TYPE dut_PMC_to_PLC :
STRUCT
	bHeartBeatMonitor	: BOOL;		

	// UI switch
	DP_sw						,
	BWR_sw						,
	DPR1_sw						,
	DPR2_sw						,
	WAT_R_sw					,
	WAT_F_sw					,
	HTR1_sw						,
	HTR2_sw						,
	HTR3_sw						,
	HTR4_sw						,
	HTR5_sw						,
	AGV_sw						,
	DEPO_sw						,
	CLN_sw						,
	T_MNT_sw					,
	T_REF_sw					,
	Pump1_ECO_sw				,
	SP1_sw						,
	PZ_sw						,
	P_CONT_sw					,
	DGZERO_sw					,
	C_EXH_sw					,
	F2_CLN_sw					,
	F_N_sw						,
	GV_AV79_Open				,
	GV_AV79_Close				,
	APC_AV71_Open				,
	APC_AV71_Close				
	: BOOL;
	
	aAV							: ARRAY[1..250] OF BOOL;	
	bAV65Open					: BOOL;
	bAV65Close					: BOOL;
	bAV79Open					: BOOL;
	bAV79Close					: BOOL;
	bAV91Open					: BOOL;
	bAV91Close					: BOOL;
	bAV202Open					: BOOL;
	bAV202Close					: BOOL;
	
	//heater
	Furnace_Temp_abnormal		: BOOL;	// Furnace temp over 1000℃
	LSC_Ht_temp_abnormal		: BOOL;	// LSC heater temperature beyond preset value
	GB_Ht_temp_abnormal			: BOOL; // Gas line heater temperature beyond preset value
	EXH_Ht_temp_abnormal		: BOOL;	// Exhaust line heater temperature beyond preset value
	CLN_Temp_abnormal			: BOOL; // furnace&exhaust line heater temperature beyond preset value
	R_Axis_Temp					: REAL;	// R axis temperature
	Inlet_Ht_1_temp				: REAL;	// Inlet heater 1 temperature
	Inlet_Ht_2_temp				: REAL;	// Inlet heater 2 temperature
	Port_Ht_1_temp				: REAL; // Port heater 1 temperature
	Port_Ht_2_temp				: REAL; // Port heater 2 temperature
	Port_Ht_3_temp				: REAL; // Port heater 3 temperature
	Port_Ht_4_temp				: REAL; // Port heater 4 temperature
	Port_Ht_5_temp				: REAL; // Port heater 5 temperature

	//Power box
	I100_00			:BOOL;	//	UPS_Fault              
	I100_01			:BOOL;	//	UPS_Alarm              
	I100_02			:BOOL;	//	UPS_Bypass_Status      
	I100_03			:BOOL;	//	UPS_Battery_Voltage_Low
	I100_04			:BOOL;	//	UPS_Start              
	I100_05			:BOOL;	//	UPS_AC_Input_Cut_Off   
	I100_06			:BOOL;	//	Powerbox_FrontDoor_sw1
	I100_07			:BOOL;	//	Powerbox_FrontDoor_sw2
	I100_08			:BOOL;	//	Powerbox_BackDoor_sw1
	I100_09			:BOOL;	//	Powerbox_BackDoor_sw2
	I100_10			:BOOL;	//	Spare11
	I100_11			:BOOL;	//	Spare12
	I100_12			:BOOL;	//	Spare13
	I100_13			:BOOL;	//	Spare14
	I100_14			:BOOL;	//	Spare15
	I100_15			:BOOL;	//	Spare16
	I101_00			:BOOL;	//	KM101_ON
	I101_01			:BOOL;	//	KM201_ON
	I101_02			:BOOL;	//	KM102_ON
	I101_03			:BOOL;	//	KM103_ON
	I101_04			:BOOL;	//	KM104_ON
	I101_05			:BOOL;	//	SPARE
	I101_06			:BOOL;	//	SPARE
	I101_07			:BOOL;	//	Furnace_Main_Breaker_Status_Monitor
	I101_08			:BOOL;	//	Blower_Breaker_Status_Feedback
	I101_09			:BOOL;	//	Zone1_Circuit_Breaker_Status_Monitor
	I101_10			:BOOL;	//	Zone2_Circuit_Breaker_Status_Monitor
	I101_11			:BOOL;	//	Zone3_Circuit_Breaker_Status_Monitor
	I101_12			:BOOL;	//	Zone4_Circuit_Breaker_Status_Monitor
	I101_13			:BOOL;	//	Zone5_Circuit_Breaker_Status_Monitor
	I101_14			:BOOL;	//	Zone6_Circuit_Breaker_Status_Monitor
	I101_15			:BOOL;	//	Zone7_Circuit_Breaker_Status_Monitor
	I102_00			:BOOL;	//	LDS1_bulk_to_process_running
	I102_01			:BOOL;	//	LDS1_supply_doing
	I102_02			:BOOL;	//	LDS1_system_ready
	I102_03			:BOOL;	//	LDS1_major_alarm
	I102_04			:BOOL;	//	LDS1_minor_alarm
	I102_05			:BOOL;	//	LDS1_low_level_status
	I102_06			:BOOL;	//	LDS1_process_reservoir_empty
	I102_07			:BOOL;	//	LDS2_bulk_to_process_running
	I102_08			:BOOL;	//	LDS2_supply_doing           
	I102_09			:BOOL;	//	LDS2_system_ready           
	I102_10			:BOOL;	//	LDS2_major_alarm            
	I102_11			:BOOL;	//	LDS2_minor_alarm            
	I102_12			:BOOL;	//	LDS2_low_level_status       
	I102_13			:BOOL;	//	LDS2_process_reservoir_empty
	I102_14			:BOOL;	//	SPARE
	I102_15			:BOOL;	//	SPARE
	I103_00			:BOOL;	//	Vaccum1_Pump_Both_On
	I103_01			:BOOL;	//	Vaccum1_Pump_Warning
	I103_02			:BOOL;	//	Vaccum1_Pump_Alarm
	I103_03			:BOOL;	//	Spare19
	I103_04			:BOOL;	//	Spare20
	I103_05			:BOOL;	//	Spare21
	I103_06			:BOOL;	//	N2_Purge_BOX_PG13_CNT1
	I103_07			:BOOL;	//	N2_Purge_BOX_PG13_CNT2
	I103_08			:BOOL;	//	N2_Purge_BOX_PG14_CNT1
	I103_09			:BOOL;	//	N2_Purge_BOX_PG14_CNT2
	I103_10			:BOOL;	//	N2_Purge_Box_PG15_CNT1
	I103_11			:BOOL;	//	N2_Purge_Box_PG15_CNT2
	I103_12			:BOOL;	//	N2_Purge_Box_PG16_CNT1
	I103_13			:BOOL;	//	N2_Purge_Box_PG16_CNT2
	I103_14			:BOOL;	//	N2_Purge_Box_PG130_CNT1
	I103_15			:BOOL;	//	N2_Purge_Box_PG130_CNT2
	I104_00			:BOOL;	//	PS17_Low_pressure_alarm
	I104_01			:BOOL;	//	Foreline_heater_light_alarm
	I104_02			:BOOL;  //	Foreline_heater_heavy_alarm
	I104_03			:BOOL;  //	Scrubber_warning
	I104_04			:BOOL;  //	Scrubber_alarm
	I104_05			:BOOL;  //	External_HPM_alarm
	I104_06			:BOOL;  //	External_EMO_In
	I104_07			:BOOL;  //	SPARE
	I104_08			:BOOL;  //	SPARE
	I104_09			:BOOL;  //	SPARE
	I104_10			:BOOL;  //	SPARE
	I104_11			:BOOL;  //	SPARE
	I104_12			:BOOL;  //	SPARE
	I104_13			:BOOL;  //	SPARE
	I104_14			:BOOL;  //	SPARE
	I104_15			:BOOL;  //	SPARE
	
	Q100_00			:BOOL;	//	VFD_RES
	Q100_01			:BOOL;	//	VFD_MRS
	Q100_02			:BOOL;	//	VFD_RT
	Q100_03			:BOOL;	//	VFD_JOG
	Q100_04			:BOOL;	//	VFD_RL
	Q100_05			:BOOL;	//	VFD_RM
	Q100_06			:BOOL;	//	VFD_RH
	Q100_07			:BOOL;	//	VFD_STP
	Q100_08			:BOOL;	//	VFD_RTR
	Q100_09			:BOOL;	//	VFD_RTF
	Q100_10			:BOOL;	//	Spare1
	Q100_11			:BOOL;	//	Spare2
	Q100_12			:BOOL;	//	Spare3
	Q100_13			:BOOL;	//	Spare4
	Q100_14			:BOOL;	//	Spare5
	Q100_15			:BOOL;	//	Spare6
	Q101_00			:BOOL;	//	Furnace 1 Zone Heating Enable
	Q101_01			:BOOL;	//	Furnace 2 Zone Heating Enable
	Q101_02			:BOOL;	//	Furnace 3 Zone Heating Enable
	Q101_03			:BOOL;	//	Furnace 4 Zone Heating Enable
	Q101_04			:BOOL;	//	Furnace 5 Zone Heating Enable
	Q101_05			:BOOL;	//	Furnace 6 Zone Heating Enable
	Q101_06			:BOOL;	//	Furnace 7 Zone Heating Enable
	Q101_07			:BOOL;	//	LSC_1_AutoRefill1 Request Or Valve Open
	Q101_08			:BOOL;	//	LSC_1_External_Shutdown
	Q101_09			:BOOL;	//	HPM Valve Out Status
	Q101_10			:BOOL;	//	Forline Heater On
	Q101_11			:BOOL;	//	Spare7
	Q101_12			:BOOL;	//	Spare8
	Q101_13			:BOOL;	//	Spare9
	Q101_14			:BOOL;	//	Spare10
	Q101_15			:BOOL;	//	Spare11
	Q102_00			:BOOL;	//	Vaccum Pump Both On
	Q102_01			:BOOL;	//	Vaccum Pump AUC On
	Q102_02			:BOOL;	//	Vaccum Pump AGV Open
	Q102_03			:BOOL;	//	LSC_2_AutoRefill1 Request Or Valve Open
	Q102_04			:BOOL;	//	LSC_2_External_Shutdown
	Q102_05			:BOOL;	//	Spare
	Q102_06			:BOOL;	//	Spare
	Q102_07			:BOOL;	//	Spare
	Q102_08			:BOOL;	//	Spare
	Q102_09			:BOOL;	//	Spare
	Q102_10			:BOOL;	//	Spare
	Q102_11			:BOOL;	//	Spare
	Q102_12			:BOOL;	//	Spare
	Q102_13			:BOOL;	//	Spare
	Q102_14			:BOOL;	//	Spare
	Q102_15			:BOOL;	//	Spare
	Q103_00			:BOOL;	//	Spare
	Q103_01			:BOOL;	//	Spare
	Q103_02			:BOOL;	//	Spare
	Q103_03			:BOOL;	//	Spare
	Q103_04			:BOOL;	//	Spare
	Q103_05			:BOOL;	//	Spare
	Q103_06			:BOOL;	//	Spare
	Q103_07			:BOOL;	//	Spare
	Q103_08			:BOOL;	//	Spare
	Q103_09			:BOOL;	//	Spare
	Q103_10			:BOOL;	//	Spare
	Q103_11			:BOOL;	//	Spare
	Q103_12			:BOOL;	//	Spare
	Q103_13			:BOOL;	//	Spare
	Q103_14			:BOOL;	//	Spare
	Q103_15			:BOOL;	//	Spare	
	
	PS17_Pressure				: REAL;	// PS17_Pressure
	
	//Gas box
	Q200_00			:BOOL;	//	OX_Pump_On
	Q200_01			:BOOL;	//	Spare1
	Q200_02			:BOOL;	//	Spare2
	Q200_03			:BOOL;	//	Spare3
	Q200_04			:BOOL;	//	Spare4
	Q200_05			:BOOL;	//	Spare5
	Q200_06			:BOOL;	//	Spare6
	Q200_07			:BOOL;	//	Spare7
	Q200_08			:BOOL;	//	Spare8
	Q200_09			:BOOL;	//	Spare9
	Q200_10			:BOOL;	//	Spare10
	Q200_11			:BOOL;	//	Spare11
	Q200_12			:BOOL;	//	Spare12
	Q200_13			:BOOL;	//	Spare13
	Q200_14			:BOOL;	//	Spare14
	Q200_15			:BOOL;	//	Spare15
	
	VG31_Reading_Valid					: BOOL;
	VG31_Overrange_Exceeded				: BOOL;
	VG31_Underrange_Exceeded			: BOOL;
	VG31_Sensor_Value					: REAL;	
	VG31_Active_Device_Warning_Details	: UDINT;
	VG31_Active_Device_Error_Details	: UDINT;
	
	//Exhaust box
	Q300_00				:BOOL;	//	CoolingValve1_Boat
	Q300_01				:BOOL;	//	CoolingValve2_Flange
	Q300_02				:BOOL;
	Q300_03				:BOOL;
	Q300_04				:BOOL;
	Q300_05				:BOOL;
	Q300_06				:BOOL;
	Q300_07				:BOOL;
	Q300_08				:BOOL;	//	APC_auto_close
	Q300_09				:BOOL;	//	APC_pump_on
	Q300_10				:BOOL;	//	BallValve_Open_Close
	Q300_11				:BOOL;
	Q300_12				:BOOL;
	Q300_13				:BOOL;
	Q300_14				:BOOL;
	Q300_15				:BOOL;

	VG11_Reading_Valid					: BOOL;
	VG11_Overrange_Exceeded				: BOOL;
	VG11_Underrange_Exceeded			: BOOL;
	VG11_Sensor_Value					: REAL;	
	VG11_Active_Device_Warning_Details	: UDINT;
	VG11_Active_Device_Error_Details	: UDINT;
	
	VG13_Reading_Valid					: BOOL;
	VG13_Overrange_Exceeded				: BOOL;
	VG13_Underrange_Exceeded			: BOOL;
	VG13_Sensor_Value					: REAL;	
	VG13_Active_Device_Warning_Details	: UDINT;
	VG13_Active_Device_Error_Details	: UDINT;
	
	VG14_Reading_Valid					: BOOL;
	VG14_Overrange_Exceeded				: BOOL;
	VG14_Underrange_Exceeded			: BOOL;
	VG14_Sensor_Value					: REAL;	
	VG14_Active_Device_Warning_Details	: UDINT;
	VG14_Active_Device_Error_Details	: UDINT;
	
	//Frontbody box
	FB_Buffer_N2_Press_Low		: BOOL;
	
	//LA box
	LA_Buffer_N2_Press_Low		: BOOL;
	Boat_at_cap_position		: BOOL;
	
	I500_00			:BOOL;	//	FIMS1_FOUP_Dock
	I500_01			:BOOL;	//	FIMS1_FOUP_Undock
	I500_02			:BOOL;	//	FIMS1_FOUP_Exist
	I500_03			:BOOL;	//	FIMS2_FOUP_Dock
	I500_04			:BOOL;	//	FIMS2_FOUP_Undock
	I500_05			:BOOL;	//	FIMS2_FOUP_Exist
	I500_06			:BOOL;	//	FIMS1_FOUP_Wafer_Shift_Detection
	I500_07			:BOOL;	//	FIMS2_FOUP_Wafer_Shift_Detection
	I500_08			:BOOL;	//	FIMS1_FOUP_Negative_Pressure
	I500_09			:BOOL;	//	FIMS1_FOUP_Ordinary_Pressure
	I500_10			:BOOL;	//	FIMS2_FOUP_Negative_Pressure
	I500_11			:BOOL;	//	FIMS2_FOUP_Ordinary_Pressure
	I500_12			:BOOL;	//	BOAT_Slow_Down_Position_Detection
	I500_13			:BOOL;	//	Buffer_Rotation_Conv_Detect_Sensor
	I500_14			:BOOL;	//	Spare1
	I500_15			:BOOL;	//	Spare2
	I501_00			:BOOL;	//	LA_Internal_Cycle_Switch_Open
	I501_01			:BOOL;	//	LA_Internal_Cycle_Switch_Close
	I501_02			:BOOL;	//	LA_ATM_Switch_Open
	I501_03			:BOOL;	//	LA_ATM_Switch_Close
	I501_04			:BOOL;	//	R-Axis_Air_Cylinder_Extend_Position
	I501_05			:BOOL;	//	R-Axis_Air_Cylinder_Retract_Position
	I501_06			:BOOL;	//	Furnace_Shutter_Open
	I501_07			:BOOL;	//	Furnace_Shutter_Close
	I501_08			:BOOL;	//	FIMS1_Exhaust_Open_Position
	I501_09			:BOOL;	//	FIMS1_Exhaust_Close_Position
	I501_10			:BOOL;	//	FIMS2_Exhaust_Open_Position
	I501_11			:BOOL;	//	FIMS2_Exhaust_Close_Position
	I501_12			:BOOL;	//	Spare3
	I501_13			:BOOL;	//	Spare4
	I501_14			:BOOL;	//	Spare5
	I501_15			:BOOL;	//	Spare6
	I502_00			:BOOL;	//	FIMS1_Seal
	I502_01			:BOOL;	//	FIMS1_Release
	I502_02			:BOOL;	//	FIMS1_Door_Close
	I502_03			:BOOL;	//	FIMS1_Door_Open
	I502_04			:BOOL;	//	FIMS1_FOUP_Latch_Off
	I502_05			:BOOL;	//	FIMS1_FOUP_Latch_On
	I502_06			:BOOL;	//	FIMS1_Collision_Avoidance_Up
	I502_07			:BOOL;	//	FIMS1_Collision_Avoidance_Down
	I502_08			:BOOL;	//	FIMS2_Seal
	I502_09			:BOOL;	//	FIMS2_Release
	I502_10			:BOOL;	//	FIMS2_Door_Close
	I502_11			:BOOL;	//	FIMS2_Door_Open
	I502_12			:BOOL;	//	FIMS2_FOUP_Latch_Off
	I502_13			:BOOL;	//	FIMS2_FOUP_Latch_On
	I502_14			:BOOL;	//	FIMS2_Collision_Avoidance_Up
	I502_15			:BOOL;	//	FIMS2_Collision_Avoidance_Down
	I503_00			:BOOL;	//	Spare7
	I503_01			:BOOL;	//	Spare8
	I503_02			:BOOL;	//	Spare9
	I503_03			:BOOL;	//	Spare10
	I503_04			:BOOL;	//	Spare11
	I503_05			:BOOL;	//	Spare12
	I503_06			:BOOL;	//	Spare13
	I503_07			:BOOL;	//	Spare14
	I503_08			:BOOL;	//	Spare15
	I503_09			:BOOL;	//	Spare16
	I503_10			:BOOL;	//	Spare17
	I503_11			:BOOL;	//	Spare18
	I503_12			:BOOL;	//	Spare19
	I503_13			:BOOL;	//	Spare20
	I503_14			:BOOL;	//	Spare21
	I503_15			:BOOL;	//	Spare22
	I504_00			:BOOL;	//	Spare23
	I504_01			:BOOL;	//	Spare24
	I504_02			:BOOL;	//	Spare25
	I504_03			:BOOL;	//	Spare26
	I504_04			:BOOL;	//	Spare27
	I504_05			:BOOL;	//	Spare28
	I504_06			:BOOL;	//	Spare29
	I504_07			:BOOL;	//	Spare30
	I504_08			:BOOL;	//	Spare31
	I504_09			:BOOL;	//	Spare32
	I504_10			:BOOL;	//	Spare33
	I504_11			:BOOL;	//	Spare34
	I504_12			:BOOL;	//	Spare35
	I504_13			:BOOL;	//	Spare36
	I504_14			:BOOL;	//	Spare37
	I504_15			:BOOL;	//	Spare38
	I505_00			:BOOL;	//	Buffer_A1_N2_Pressure_Alarm
	I505_01			:BOOL;	//	Buffer_A1_FOUP_Detect
	I505_02			:BOOL;	//	Buffer_B1_N2_Pressure_Alarm
	I505_03			:BOOL;	//	Buffer_B1_FOUP_Detect
	I505_04			:BOOL;	//	Buffer_C1_N2_Pressure_Alarm
	I505_05			:BOOL;	//	Buffer_C1_FOUP_Detect
	I505_06			:BOOL;	//	Buffer_D1_N2_Pressure_Alarm
	I505_07			:BOOL;	//	Buffer_D1_FOUP_Detect
	I505_08			:BOOL;	//	Buffer_A2_N2_Pressure_Alarm
	I505_09			:BOOL;	//	Buffer_A2_FOUP_Detect
	I505_10			:BOOL;	//	Buffer_B2_N2_Pressure_Alarm
	I505_11			:BOOL;	//	Buffer_B2_FOUP_Detect
	I505_12			:BOOL;	//	Buffer_C2_N2_Pressure_Alarm
	I505_13			:BOOL;	//	Buffer_C2_FOUP_Detect
	I505_14			:BOOL;	//	Buffer_D2_N2_Pressure_Alarm
	I505_15			:BOOL;	//	Buffer_D2_FOUP_Detect
	I506_00			:BOOL;	//	Buffer_A3_N2_Pressure_Alarm
	I506_01			:BOOL;	//	Buffer_A3_FOUP_Detect
	I506_02			:BOOL;	//	Buffer_B3_N2_Pressure_Alarm
	I506_03			:BOOL;	//	Buffer_B3_FOUP_Detect
	I506_04			:BOOL;	//	Buffer_C3_N2_Pressure_Alarm
	I506_05			:BOOL;	//	Buffer_C3_FOUP_Detect
	I506_06			:BOOL;	//	Buffer_D3_N2_Pressure_Alarm
	I506_07			:BOOL;	//	Buffer_D3_FOUP_Detect
	I506_08			:BOOL;	//	Buffer_A4_N2_Pressure_Alarm
	I506_09			:BOOL;	//	Buffer_A4_FOUP_Detect
	I506_10			:BOOL;	//	Buffer_B4_N2_Pressure_Alarm
	I506_11			:BOOL;	//	Buffer_B4_FOUP_Detect
	I506_12			:BOOL;	//	Buffer_C4_N2_Pressure_Alarm
	I506_13			:BOOL;	//	Buffer_C4_FOUP_Detect
	I506_14			:BOOL;	//	Buffer_D4_N2_Pressure_Alarm
	I506_15			:BOOL;	//	Buffer_D4_FOUP_Detect
	
	Q500_00			:BOOL;	//	LA_Internal_Air_Cycle_Switch_Open
	Q500_01			:BOOL;	//	LA_Internal_Air_Cycle_Switch_Close
	Q500_02			:BOOL;	//	LA_ATM_Switch_Open
	Q500_03			:BOOL;	//	LA_ATM_Switch_Close
	Q500_04			:BOOL;	//	R_Axis_Air_Cylinder_Extend_Switch
	Q500_05			:BOOL;	//	R_Axis_Air_Cylinder_Retract_Switch
	Q500_06			:BOOL;	//	O2_Detector_Switch_LA_POD
	Q500_07			:BOOL;	//	O2_Detector_Switch_POD1_POD2
	Q500_08			:BOOL;	//	LA_Internal_Air_Cycle_Fan1_Switch
	Q500_09			:BOOL;	//	LA_Internal_Air_Cycle_Fan2_Switch
	Q500_10			:BOOL;	//	LA_Internal_Air_Cycle_Fan3_Switch
	Q500_11			:BOOL;	//	LA_Internal_Air_Cycle_Fan4_Switch
	Q500_12			:BOOL;	//	Furnace_Shutter_Open
	Q500_13			:BOOL;	//	Furnace_Shutter_Close
	Q500_14			:BOOL;	//	Spare1
	Q500_15			:BOOL;	//	Spare2
	Q501_00			:BOOL;	//	POD1_Exhaust_Switch_Open
	Q501_01			:BOOL;	//	POD1_Exhaust_Switch_Close
	Q501_02			:BOOL;	//	POD2_Exhaust_Switch_Open
	Q501_03			:BOOL;	//	POD2_Exhaust_Switch_Close
	Q501_04			:BOOL;	//	Spare3
	Q501_05			:BOOL;	//	Spare4
	Q501_06			:BOOL;	//	Spare5
	Q501_07			:BOOL;	//	Spare6
	Q501_08			:BOOL;	//	Spare7
	Q501_09			:BOOL;	//	Spare8
	Q501_10			:BOOL;	//	Spare9
	Q501_11			:BOOL;	//	Spare10
	Q501_12			:BOOL;	//	Spare11
	Q501_13			:BOOL;	//	Spare12
	Q501_14			:BOOL;	//	Spare13
	Q501_15			:BOOL;	//	Spare14
	Q502_00			:BOOL;	//	Buffer_A1_N2_Purge_Switch
	Q502_01			:BOOL;	//	Buffer_B1_N2_Purge_Switch
	Q502_02			:BOOL;	//	Buffer_C1_N2_Purge_Switch
	Q502_03			:BOOL;	//	Buffer_D1_N2_Purge_Switch
	Q502_04			:BOOL;	//	Buffer_A2_N2_Purge_Switch
	Q502_05			:BOOL;	//	Buffer_B2_N2_Purge_Switch
	Q502_06			:BOOL;	//	Buffer_C2_N2_Purge_Switch
	Q502_07			:BOOL;	//	Buffer_D2_N2_Purge_Switch
	Q502_08			:BOOL;	//	Buffer_A3_N2_Purge_Switch
	Q502_09			:BOOL;	//	Buffer_B3_N2_Purge_Switch
	Q502_10			:BOOL;	//	Buffer_C3_N2_Purge_Switch
	Q502_11			:BOOL;	//	Buffer_D3_N2_Purge_Switch
	Q502_12			:BOOL;	//	Buffer_A4_N2_Purge_Switch
	Q502_13			:BOOL;	//	Buffer_B4_N2_Purge_Switch
	Q502_14			:BOOL;	//	Buffer_C4_N2_Purge_Switch
	Q502_15			:BOOL;	//	Buffer_D4_N2_Purge_Switch
	Q503_00			:BOOL;
	Q503_01         :BOOL;
	Q503_02         :BOOL;
	Q503_03         :BOOL;
	Q503_04         :BOOL;
	Q503_05         :BOOL;
	Q503_06         :BOOL;
	Q503_07         :BOOL;
	Q503_08         :BOOL;
	Q503_09         :BOOL;
	Q503_10         :BOOL;
	Q503_11         :BOOL;
	Q503_12         :BOOL;
	Q503_13         :BOOL;
	Q503_14         :BOOL;
	Q503_15	        :BOOL;
	
	//Safety box
	O2_analyzer_over_range_alarm		,
	SCR_ONOFF_SWITCH					,
	O2_analyzer_fault					,
	SMK1_detector_operator				,
	SMK1_detector_fault					,
	SMK1_detector_fire_alarm			,
	GD201_NF3_gas_leak_1st_alarm		,
	GD201_NF3_gas_leak_2nd_alarm		,
	GD202_SiH4_gas_leak_1st_alarm		,
	GD201_fault							,
	GD202_SiH4_gas_leak_2nd_alarm		,
	GD202_fault							,
	GD203_NH3_gas_leak_2nd_alarm		,
	GD203_NH3_gas_leak_1st_alarm		,
	GD203_fault							,
	GD204_HCL_gas_leak_1st_alarm		,
	GD204_fault							,
	GD204_HCL_gas_leak_2nd_alarm		,
	GD205_F2_gas_leak_1st_alarm			,
	GD205_F2_gas_leak_2nd_alarm			,
	GD206_NF3_gas_leak_1st_alarm		,
	GD205_fault							,
	GD206_NF3_gas_leak_2nd_alarm		,
	GD206_fault							,
	GD207_SiH4_gas_leak_2nd_alarm		,
	GD207_SiH4_gas_leak_1st_alarm		,
	GD207_fault							,
	GD208_NH3_gas_leak_1st_alarm		,
	GD208_fault							,
	GD208_NH3_gas_leak_2nd_alarm		,
	GD209_HCL_gas_leak_1st_alarm		,
	GD209_HCL_gas_leak_2nd_alarm		,
	GD210_F2_gas_leak_1st_alarm			,
	GD209_fault							,
	GD210_F2_gas_leak_2nd_alarm			,
	GD210_fault							,
	TS31_Cap_outside_temp_sw			,
	TS30_Cap_inside_temp_sw				,
	TS34_R_axis_rotation_temp_sw		,
	Loading_area_EMS					,
	SL201_gas_box_door_sw1_1			,
	FFU_temp_sw							,
	SL201_gas_box_door_sw1_2			,
	SL202_gas_box_door_sw2_1			,
	SL203_gas_box_door_sw3_1			,
	SL202_gas_box_door_sw2_2			,
	SL203_gas_box_door_sw3_2			,
	SL204_gas_box_door_sw4_1			,
	SL205_gas_box_door_sw5_1			,
	SL204_gas_box_door_sw4_2			,
	SL205_gas_box_door_sw5_2			,
	SL501_LA_door_sw1					,
	SL503_LA_door_sw3					,
	SL502_LA_door_sw2					,
	SL504_furnace_door_sw				,
	Gas_box_exhaust_pressure_alarm_1st	,
	MS2_S_gas_box_exhaust_alarm			,
	Gas_box_exhaust_pressure_alarm_2nd	,
	MS11_S_gas_box_exhaust_alarm		,
	MS12_S_gas_box_exhaust_alarm		,
	LSC_1_leak_alarm					,
	LD501_Magnetic_fluid_leak			,
	LD502_Cooling_water_leak			,
	TS305_RHC_temp_sw					,
	LD503_RHC_leak						,
	TS306_Main_furnace_Temp_sw			,
	LD301_water_leak_alarm				,
	EMO301_Exhaust_box_EMO				,
	LD302_water_leak_alarm				,
	FS101_water_flow_alarm1				,	//水路总流量
	Buffer_motor_EDM					,
	R_axis_motor_EDM					,
	E_axis_motor_EDM					,
	FS101_water_flow_alarm2				,	//水路总流量
	EMO101_power_box_EMO				,
	Furnace_transformer_temp_sw			,
	Power_box_fire_detector_alarm		,
	AC100V_transformer_temp_sw			,
	Furnace_power_on_switch				,
	Power_box_reset_button				,
	AC100V_transformer_power_on_switch	,
	VFD_EDM								,
	Light_curtain_fault					,
	Light_curtain_OSSD2					,
	Light_curtain_OSSD1					,
	Gas_box_reset_button				,
	EMO401_frontbody_EMO				,
	Frontbody_IO_shutter				,
	Frontbody_door_sw					,
	Frontbody_reset_button	
	:BOOL;
	
	//IO mapping
	HPM_valve_power_on_off				,
	Furnace_power_on					,
	Cap_heater_enable					,
	//spare
	AC100V_transformer_power_on			,
	VFD_Enable							,
	Blower_power_on						,
	Buffer_motor_enable1				,
	Buffer_motor_enable2				,
	Boat_motor_enable2					,
	Boat_motor_enable1					,
	FTR_enable1							,
	FTR_enable2							,
	WTR_enable1							,
	FTR_interlock_reset					,
	WTR_enable2							,
	WTR_interlock_reset					,
	R_axis_motor_enable2				,
	R_axis_motor_enable1				,
	//spare
	//spare
	Light_curtain_idle					,
	//spare
	Frontbody_interlock_indicator		,
	GasBox_interlock_indicator
	: BOOL;
	
	//FFU
	FFU_ALARM_EN	:	REAL;	//报警输出使能
	FFU_HSPEED		:	REAL;	//转速上限
	FFU_LSPEED		:	REAL;	//转速下限
	
	FFU1_1_POWER_ON	:	REAL	;	//	0:停止，1：运行
	FFU1_2_POWER_ON	:	REAL	;	//	0:停止，1：运行
	FFU1_3_POWER_ON	:	REAL	;	//	0:停止，1：运行
	FFU1_4_POWER_ON	:	REAL	;	//	0:停止，1：运行
	FFU1_5_POWER_ON	:	REAL	;	//	0:停止，1：运行
	FFU1_6_POWER_ON	:	REAL	;	//	0:停止，1：运行
	FFU2_1_POWER_ON	:	REAL	;	//	0:停止，1：运行
	FFU2_2_POWER_ON	:	REAL	;	//	0:停止，1：运行
	FFU2_3_POWER_ON	:	REAL	;	//	0:停止，1：运行
	FFU2_4_POWER_ON	:	REAL	;	//	0:停止，1：运行
	FFU2_5_POWER_ON	:	REAL	;	//	0:停止，1：运行
	FFU2_6_POWER_ON	:	REAL	;	//	0:停止，1：运行
	FFU3_1_POWER_ON	:	REAL	;	//	0:停止，1：运行
	FFU3_2_POWER_ON	:	REAL	;	//	0:停止，1：运行
	FFU3_3_POWER_ON	:	REAL	;	//	0:停止，1：运行
	FFU3_4_POWER_ON	:	REAL	;	//	0:停止，1：运行
	FFU3_5_POWER_ON	:	REAL	;	//	0:停止，1：运行
	FFU3_6_POWER_ON	:	REAL	;	//	0:停止，1：运行
	
	FFU1_1_SPEED_SV	:	REAL	;	//	FFU1_1设定转速
	FFU1_2_SPEED_SV	:	REAL	;	//	FFU1_2设定转速
	FFU1_3_SPEED_SV	:	REAL	;	//	FFU1_3设定转速
	FFU1_4_SPEED_SV	:	REAL	;	//	FFU1_4设定转速
	FFU1_5_SPEED_SV	:	REAL	;	//	FFU1_5设定转速
	FFU1_6_SPEED_SV	:	REAL	;	//	FFU1_6设定转速
	FFU2_1_SPEED_SV	:	REAL	;	//	FFU2_1设定转速
	FFU2_2_SPEED_SV	:	REAL	;	//	FFU2_2设定转速
	FFU2_3_SPEED_SV	:	REAL	;	//	FFU2_3设定转速
	FFU2_4_SPEED_SV	:	REAL	;	//	FFU2_4设定转速
	FFU2_5_SPEED_SV	:	REAL	;	//	FFU2_5设定转速
	FFU2_6_SPEED_SV	:	REAL	;	//	FFU2_6设定转速
	FFU3_1_SPEED_SV	:	REAL	;	//	FFU3_1设定转速
	FFU3_2_SPEED_SV	:	REAL	;	//	FFU3_2设定转速
	FFU3_3_SPEED_SV	:	REAL	;	//	FFU3_3设定转速
	FFU3_4_SPEED_SV	:	REAL	;	//	FFU3_4设定转速
	FFU3_5_SPEED_SV	:	REAL	;	//	FFU3_5设定转速
	FFU3_6_SPEED_SV	:	REAL	;	//	FFU3_6设定转速
	
	FFU1_1_EN		:	REAL	;	//	FFU1_1使能
	FFU1_2_EN		:	REAL	;	//	FFU1_2使能
	FFU1_3_EN		:	REAL	;	//	FFU1_3使能
	FFU1_4_EN		:	REAL	;	//	FFU1_4使能
	FFU1_5_EN		:	REAL	;	//	FFU1_5使能
	FFU1_6_EN		:	REAL	;	//	FFU1_6使能
	FFU2_1_EN		:	REAL	;	//	FFU2_1使能
	FFU2_2_EN		:	REAL	;	//	FFU2_2使能
	FFU2_3_EN		:	REAL	;	//	FFU2_3使能
	FFU2_4_EN		:	REAL	;	//	FFU2_4使能
	FFU2_5_EN		:	REAL	;	//	FFU2_5使能
	FFU2_6_EN		:	REAL	;	//	FFU2_6使能
	FFU3_1_EN		:	REAL	;	//	FFU3_1使能
	FFU3_2_EN		:	REAL	;	//	FFU3_2使能
	FFU3_3_EN		:	REAL	;	//	FFU3_3使能
	FFU3_4_EN		:	REAL	;	//	FFU3_4使能
	FFU3_5_EN		:	REAL	;	//	FFU3_5使能
	FFU3_6_EN		:	REAL	;	//	FFU3_6使能
		
END_STRUCT
END_TYPE
